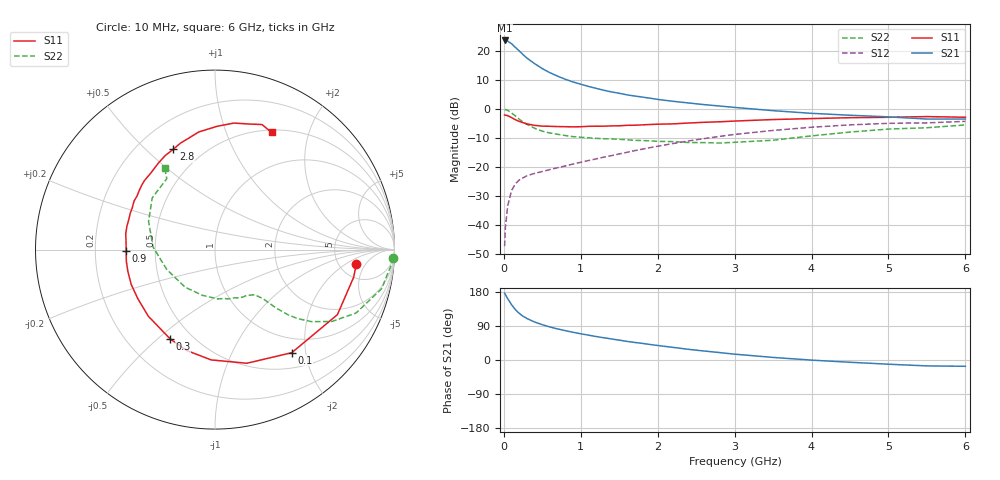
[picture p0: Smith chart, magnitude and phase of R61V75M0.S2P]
! SIEMENS Small Signal Semiconductors
! BFR193
! Si NPN RF Bipolar Junction Transistor in SOT23
! VCE = 1.75 V  IC = 5 mA
! Common Emitter S-Parameters:  May  1996
# GHz  S  MA  R  50
!  f  S11  S21  S12  S22
! GHz  MAG  ANG  MAG  ANG  MAG  ANG  MAG  ANG
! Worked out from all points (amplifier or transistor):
!   36 points, 10 MHz to 6 GHz, reference 50 ohm
!   highest |S21| = 23.7 dB at 10 MHz (marker M1)
!   |S21| within 3 dB of that: start of sweep to 174.9 MHz
!   unconditionally stable (mu >= 1): 881.2 MHz to 2.026 GHz
!   at 250 MHz: K = 0.43, MSG = 21.3 dB, |S12| = -23.7 dB
!   at 1.4 GHz: K = 1.07, MAG = 9.4 dB, |S12| = -16.0 dB
!   at 6 GHz: K = 0.97, MSG = 0.4 dB, |S12| = -4.2 dB
!   S11 on the Smith chart (normalised r, x): 10 MHz: 7.23, -3.09; 100 MHz: 0.74, -1.75; 300 MHz: 0.38, -0.55; 900 MHz: 0.34, -0.01; 2.8 GHz: 0.35, +0.61; 6 GHz: 0.53, +1.46
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0.01  0.7911 -5.8  15.38 176.6  0.0043 85.7  0.9909 -2.6
0.02  0.788 -11.2  15.15 172.6  0.009 82.9  0.9836 -5.4
0.05  0.7724 -28.0  14.98 161.8  0.0213 76.5  0.9534 -13.2
0.1  0.7162 -53.3  13.5 146.1  0.0392 65.1  0.8619 -24.2
0.15  0.6577 -74.3  11.65 132.8  0.0515 57.2  0.7644 -31.6
0.2  0.615 -92.0  10.16 123.1  0.0597 52.0  0.6718 -36.7
0.25  0.5835 -105.9  8.733 115.4  0.0651 48.9  0.5988 -39.9
0.3  0.5563 -116.8  7.635 109.5  0.0708 47.1  0.5476 -41.7
0.4  0.5251 -135.1  6.12 100.3  0.0777 45.8  0.4679 -43.8
0.5  0.5096 -147.5  5.015 93.1  0.0837 46.8  0.4162 -44.8
0.6  0.5056 -157.4  4.257 87.1  0.0906 47.6  0.3874 -45.5
0.7  0.5005 -165.9  3.714 81.9  0.0974 49.1  0.3674 -46.5
0.9  0.4948 -179.2  2.949 73.1  0.1128 52.4  0.3354 -48.8
1.1  0.5053 169.9  2.473 65.6  0.1296 55.1  0.3197 -52.7
1.3  0.5086 160.8  2.122 58.7  0.1485 56.4  0.3085 -56.9
1.6  0.5257 149.0  1.768 49.1  0.1796 57.5  0.2961 -65.3
2.2  0.5572 129.7  1.367 33.3  0.2548 55.3  0.2752 -86.9
2.8  0.6052 112.6  1.135 19.7  0.3379 48.8  0.2602 -117.1
3.5  0.6618 97.8  0.942 6.8  0.4294 38.0  0.2906 -157.5
4.5  0.7129 81.5  0.785 -6.0  0.5355 21.2  0.402 157.0
5.5  0.7443 69.4  0.675 -15.6  0.5796 4.4  0.4778 124.2
6  0.725 64.2  0.675 -16.6  0.6157 -0.4  0.5341 121.7
